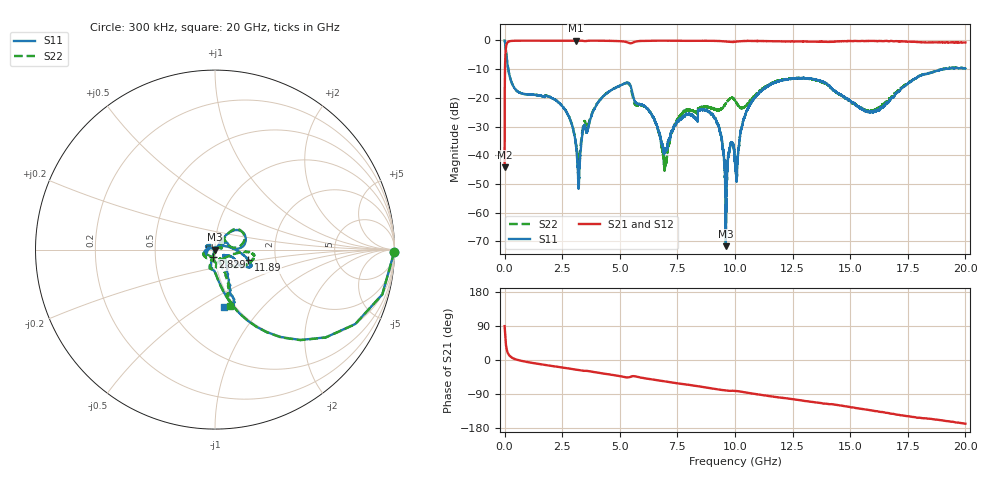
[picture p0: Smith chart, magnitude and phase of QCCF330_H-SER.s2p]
!{QCCF330}
!Johanson Technology Inc.
!www.johansontechnology.com
!Test Board Conditions:
!Substrate Type  RO4350B
!Substrate Thickness  10 mil
!Substrate Dk  3.66
!TL Type: GCPW
!TL Trace Width  21 mil
!TL Gap  20 mil
!Electrode orientation  Horizontal
!DUT TOPOLOGY	SERIES
!Mounting Pad LxW  16x21 mil
! Created Sat Jan  9 18:22:06 2021
# hz S ma R 50
! 2 Port Network Data from SP1.SP block
! freq  magS11  angS11  magS21  angS21  magS12  angS12  magS22  angS22
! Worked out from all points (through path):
!   20001 points, 300 kHz to 20 GHz, reference 50 ohm
!   highest |S21| = -0.04 dB at 3.095 GHz (marker M1); lowest = -44.2 dB at 300 kHz (marker M2)
!   group delay of S21, straight-line fit = 24 ps
!   lowest |S11| = -71.7 dB at 9.6 GHz (marker M3), VSWR 1.00, Z = 50 - j0.000798 ohm
!   |S11| at or under -10 dB: 156.3 MHz to 19.11 GHz (18.95 GHz wide, 197 % of centre)
!   |S22| runs from -45.4 to 0.0 dB; largest |S21 - S12| = 0.013
!   S11 on the Smith chart (normalised r, x): 300 kHz: open; 2.829 GHz: 0.97, -0.08; 11.89 GHz: 1.44, -0.18; 20 GHz: 0.89, -0.64
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300000  0.9986 -0.7  0.006148 89.4  0.005953 88.7  0.9995 -0.6
1.023e8  0.4456 -64.6  0.8919 25.3  0.8934 25.2  0.4456 -64.5
1.673e8  0.2984 -74.4  0.9519 15.2  0.9528 15.2  0.2979 -74.5
2.8293e9  0.04352 -108.3  0.995 -22.7  0.9938 -22.7  0.04332 -108.3
3.0953e9  0.01526 -105.6  0.9953 -25.2  0.9936 -25.2  0.01608 -91.8
3.2143e9  0.002871 -40.7  0.9939 -26.4  0.9929 -26.4  0.008364 -26.7
3.3343e9  0.01656 41.2  0.9896 -27.6  0.9897 -27.6  0.02016 25.8
4.0643e9  0.08364 54.6  0.9894 -33.6  0.9895 -33.6  0.0846 50.7
5.2783e9  0.1839 30.8  0.9399 -45.7  0.9396 -45.7  0.1802 33.5
6.6673e9  0.02763 42.7  0.9905 -53.8  0.991 -53.9  0.02653 40.8
6.9693e9  0.01189 111.0  0.9913 -56.7  0.9924 -56.7  0.006396 -46.5
7.6903e9  0.04261 165.3  0.9831 -63.1  0.985 -63.2  0.052 -101.8
8.8433e9  0.05683 -169.6  0.9857 -73.4  0.9849 -73.4  0.06841 -145.7
9.3363e9  0.02641 161.6  0.9755 -78.3  0.9763 -78.4  0.06181 -107.3
9.6003e9  0.0002596 -1.8  0.9579 -80.6  0.9575 -80.6  0.07951 -83.5
9.8243e9  0.01668 -82.0  0.9398 -81.4  0.9387 -81.4  0.1003 -82.6
1.00003e10  0.007621 -141.2  0.9502 -81.3  0.9474 -81.4  0.08975 -86.6
1.06003e10  0.06901 14.3  0.9808 -87.0  0.9825 -87.0  0.08284 -27.0
1.18863e10  0.1941 -17.7  0.9639 -98.6  0.9631 -98.6  0.1991 -4.4
1.33343e10  0.2144 -27.5  0.9536 -110.5  0.9549 -110.7  0.2113 -18.0
1.66673e10  0.08448 -48.6  0.9681 -140.2  0.9727 -140.5  0.09486 -68.1
2e10  0.3245 -81.0  0.9232 -168.0  0.9192 -168.0  0.3267 -75.5
